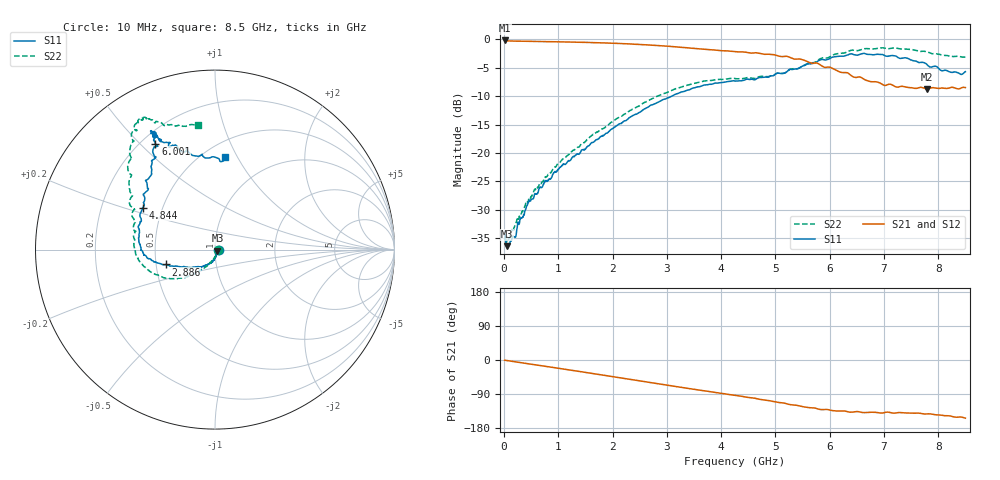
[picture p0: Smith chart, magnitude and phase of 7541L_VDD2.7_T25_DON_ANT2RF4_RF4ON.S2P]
!Agilent Technologies,E5071C,MY46417908,A.11.23
!Date: Wed Dec 09 17:18:32 2020
!Data & Calibration Information:
!Freq	S11:SOLT2(ON)	S21:SOLT2(ON)	S12:SOLT2(ON)	S22:SOLT2(ON)
!PortZ  Port1:50+j0  Port2:50+j0
!Above PortZ is port z conversion or system Z0 setting when saving the data.
!When reading, reference impedance value at option line is always used.
# Hz S dB R 50
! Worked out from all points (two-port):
!   1601 points, 10 MHz to 8.5 GHz, reference 50 ohm
!   highest |S21| = -0.20 dB at 10 MHz (marker M1); lowest = -8.8 dB at 7.794 GHz (marker M2)
!   |S21| within 3 dB of the highest: start of sweep to 5.267 GHz
!   lowest |S11| = -36.4 dB at 47.14 MHz (marker M3), VSWR 1.03, Z = 51.4 - j0.659 ohm
!   |S11| at or under -10 dB: start of sweep to 3.091 GHz
!   |S22| runs from -35.8 to -1.5 dB; largest |S21 - S12| = 0.0037
!   S11 on the Smith chart (normalised r, x): 10 MHz: 1.04, -0.00; 2.886 GHz: 0.56, -0.10; 4.844 GHz: 0.39, +0.23; 6.001 GHz: 0.25, +0.56; 8.5 GHz: 0.63, +0.89
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1e7  -33.94 -2.2  -0.20 -0.5  -0.20 -0.5  -35.04 -13.0
4.714375e7  -36.39 -25.0  -0.27 -1.3  -0.27 -1.3  -35.50 -26.1
7.898125e7  -35.99 -34.4  -0.28 -2.0  -0.28 -2.0  -35.54 -36.3
1.798e8  -34.73 -53.1  -0.31 -4.2  -0.32 -4.2  -33.18 -55.4
4.345e8  -29.03 -79.2  -0.36 -9.7  -0.36 -9.7  -28.69 -85.4
5.724625e8  -27.15 -86.0  -0.38 -12.6  -0.38 -12.6  -26.39 -95.2
1.060638e9  -22.33 -106.8  -0.45 -23.1  -0.45 -23.1  -21.27 -111.9
1.426769e9  -19.49 -122.2  -0.53 -31.1  -0.53 -31.1  -18.39 -121.2
2.164338e9  -14.75 -147.6  -0.74 -47.5  -0.74 -47.5  -13.53 -135.1
2.843538e9  -11.04 -162.3  -1.11 -62.8  -1.11 -62.8  -9.93 -150.2
2.885988e9  -10.82 -163.2  -1.13 -63.7  -1.14 -63.8  -9.78 -151.0
3.681925e9  -8.06 -175.5  -1.76 -81.3  -1.76 -81.2  -7.34 -172.1
4.255e9  -7.34 170.9  -2.18 -93.2  -2.17 -93.2  -6.90 174.9
4.843994e9  -6.66 149.7  -2.62 -106.2  -2.61 -106.2  -6.58 161.2
5.252575e9  -5.33 135.4  -3.13 -117.2  -3.13 -117.2  -5.37 152.0
5.671769e9  -4.28 122.6  -4.22 -126.0  -4.18 -126.0  -4.12 138.5
6.000756e9  -3.38 119.3  -4.91 -132.0  -4.92 -132.0  -3.07 132.1
6.430562e9  -2.65 117.7  -6.60 -137.4  -6.61 -137.2  -1.90 124.0
7.088538e9  -2.93 118.4  -7.90 -137.9  -7.93 -138.0  -1.65 119.3
7.428138e9  -3.32 117.0  -8.45 -139.8  -8.46 -139.6  -1.74 117.4
7.794269e9  -4.48 109.9  -8.77 -142.2  -8.80 -142.2  -2.22 113.4
8.5e9  -5.69 83.6  -8.49 -153.5  -8.55 -153.5  -3.09 97.7
